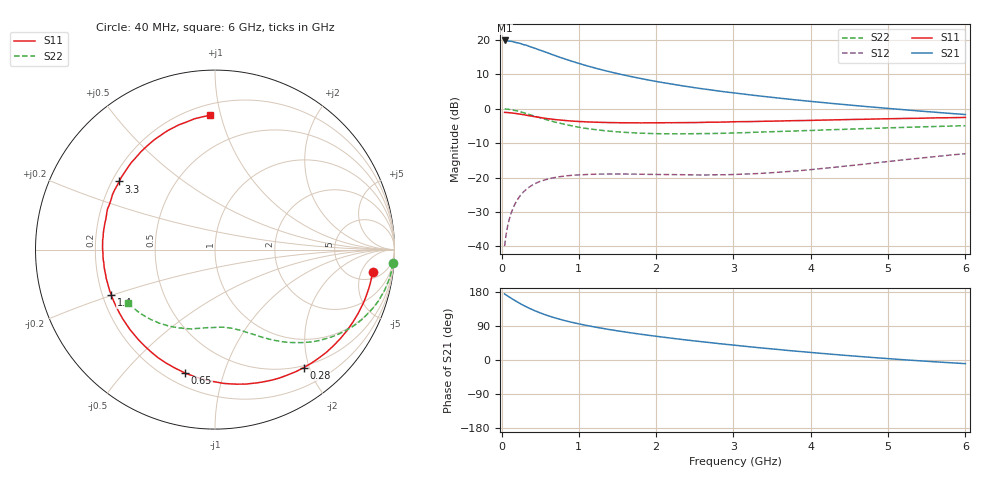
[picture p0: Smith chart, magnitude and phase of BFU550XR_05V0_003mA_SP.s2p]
! Filename:  P:\Prog\Test\Noise\ATS_data\Testdata_Net\03 Spar\BFU550XR_APG2013_45_C05_05p0V_003mA_SP_CM01_D.s2p
! Date/Time: Tue 06/Aug/2013 14:38:15
! BFU550XR_APG2013_45_C05_05p0V_1to35mA_SP_CM01_Bias3_R.s2p
! MDIF S-parameter v. bias file
! BFU550XR_APG2013_45_C05_05p0V_1to35mA_SP_CM01
! Date/time Fri Aug 02 14:46:46 2013
! VAR V_out= 5.0000
! VAR I_out= 3.0050
! VAR V_in= 0.8024
! VAR I_in= 0.0326
! Device data file deembeded for feedlines and parallel
! Original file: \03 Spar\BFU550XR_APG2013_45_C05_05p0V_003mA_SP_CM01_R.s2p
! Feed-files: PR006V01_02082013_Feed1.s2p, PR006V01_02082013_Feed2.s2p
! Parallel-file: PR006V01_02082013_Par.s2p
# MHz S MA R 50
!  Freq-MHz  S11-mag  S11-arg  S21-mag  S21-arg  S12-mag  S12-arg  S22-mag  S22-arg
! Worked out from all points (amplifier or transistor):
!   98 points, 40 MHz to 6 GHz, reference 50 ohm
!   highest |S21| = 19.9 dB at 40 MHz (marker M1)
!   |S21| within 3 dB of that: start of sweep to 520.9 MHz
!   unconditionally stable (mu >= 1): 2.764 GHz to 4.487 GHz
!   at 300 MHz: K = 0.13, MSG = 21.2 dB, |S12| = -23.9 dB
!   at 1.6 GHz: K = 0.61, MSG = 14.4 dB, |S12| = -19.0 dB
!   at 6 GHz: K = 0.82, MSG = 5.7 dB, |S12| = -13.1 dB
!   S11 on the Smith chart (normalised r, x): 40 MHz: 7, -8; 280 MHz: 0.47, -1.91; 650 MHz: 0.27, -0.75; 1.4 GHz: 0.24, -0.20; 3.3 GHz: 0.23, +0.30; 6 GHz: 0.27, +0.93
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40  0.8878 -8.1  9.876 174.5  0.01004 85.0  0.9944 -4.4
50  0.8863 -10.0  9.872 172.4  0.01244 84.3  0.9922 -5.6
140  0.8679 -27.8  9.519 161.0  0.03379 74.1  0.9621 -15.5
220  0.8438 -42.8  9.078 151.4  0.05037 66.0  0.9187 -23.4
280  0.823 -53.0  8.608 144.7  0.06109 60.5  0.8816 -28.8
320  0.8068 -60.1  8.417 140.4  0.06723 57.2  0.854 -32.1
440  0.7656 -78.2  7.544 129.3  0.08225 48.6  0.7763 -40.5
550  0.7317 -92.6  6.814 120.5  0.09167 42.2  0.7101 -46.9
650  0.708 -103.6  6.184 113.8  0.09827 37.6  0.6619 -51.4
750  0.6881 -113.4  5.639 107.8  0.1028 33.9  0.6192 -55.3
850  0.6718 -122.3  5.176 102.4  0.1062 30.7  0.5831 -58.8
1050  0.6503 -136.7  4.404 93.2  0.1099 26.0  0.5282 -64.5
1200  0.6397 -145.8  3.949 87.3  0.1117 23.4  0.5003 -68.0
1400  0.6304 -156.3  3.461 80.2  0.1125 20.9  0.4729 -72.3
1700  0.625 -169.2  2.911 70.9  0.112 18.9  0.4473 -78.2
2050  0.6268 178.5  2.446 61.3  0.1107 18.3  0.4344 -84.3
2500  0.631 164.9  2.029 50.3  0.1095 19.9  0.4348 -92.0
3100  0.6506 149.3  1.655 37.2  0.1119 25.4  0.4483 -101.8
3300  0.6549 144.6  1.555 33.0  0.1142 27.3  0.4575 -105.1
4100  0.6836 127.3  1.252 18.1  0.1339 34.4  0.4887 -118.1
5200  0.7239 106.0  0.9714 0.7  0.1812 36.4  0.5363 -135.7
6000  0.7494 92.1  0.8259 -9.6  0.2223 32.9  0.5685 -148.2
